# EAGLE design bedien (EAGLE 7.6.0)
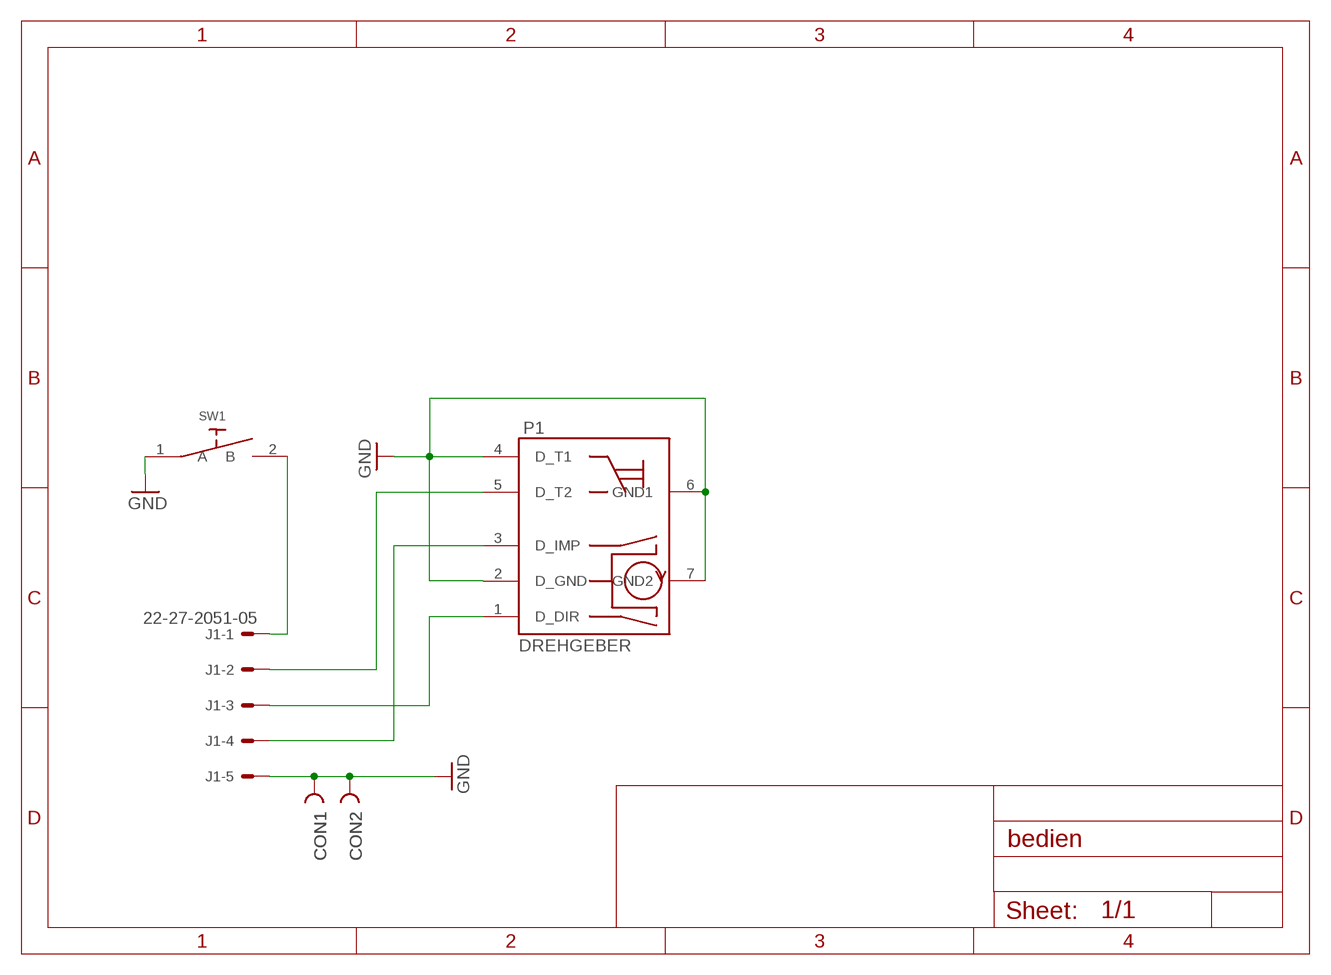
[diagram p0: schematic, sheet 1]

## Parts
CON1  PIN2_53MM  [HOLE3]
CON2  PIN2_53MM  [HOLE3]
J1  22-27-2051-05  [6410-05]
P1  DREHGEBER  [DREHG]
SW1  MTG-TASTER  [MTG]

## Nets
GND: CON1.1 CON2.1 J1.5 P1.2(D_GND) P1.4(D_T1) P1.6(GND1) P1.7(GND2) SW1.1(A)
N$1: J1.3 P1.1(D_DIR)
N$2: J1.4 P1.3(D_IMP)
N$3: J1.2 P1.5(D_T2)
N$4: J1.1 SW1.2(B)

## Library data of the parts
CON1 CON2 = lindenau:PIN2_5
J1 = con-molex:22-?-05: CONNECTOR wire to board 2.54 mm (.1 inch) pitch header; OC_FARNELL: unknown; OC_NEWARK: unknown
P1 = lindenau:DREHGEBER
SW1 = lindenau:MTG-TASTER

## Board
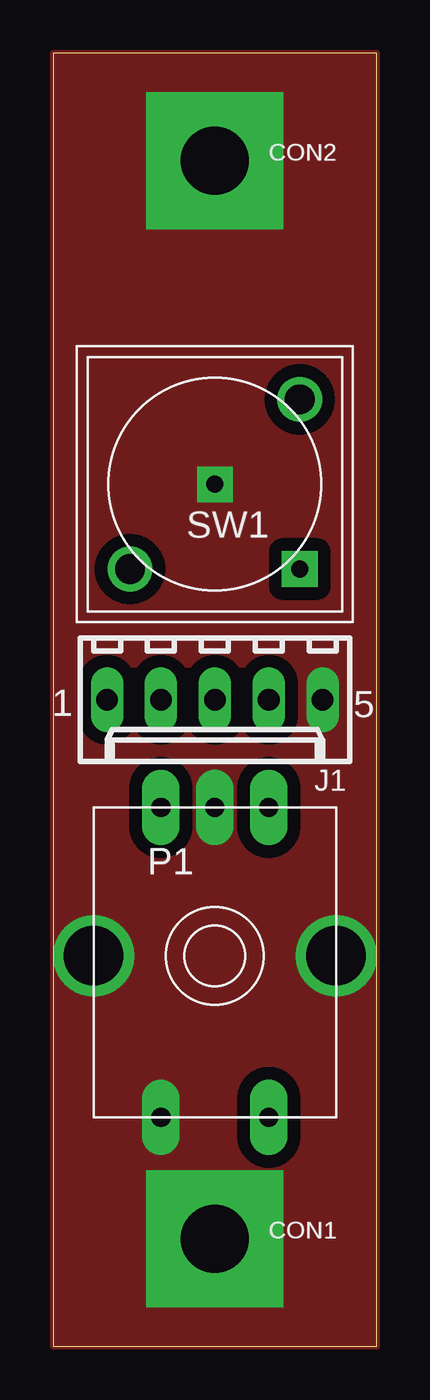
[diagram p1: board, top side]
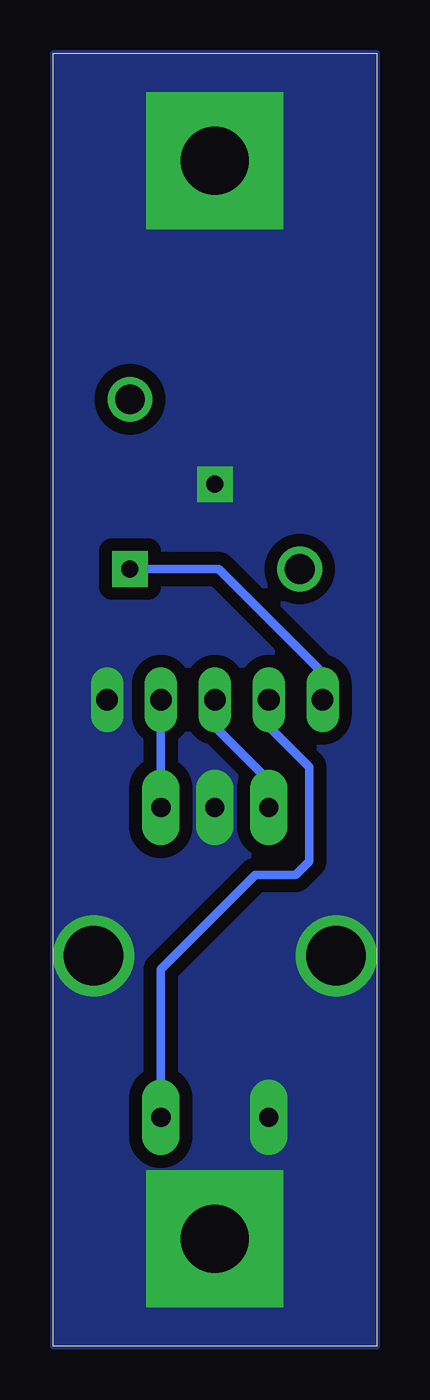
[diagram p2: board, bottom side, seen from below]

Size 15.24 x 60.96 mm. Coordinates in mm from the lower left corner, seen from the top.
Outline: 0,60.96 0,0 15.24,0 15.24,60.96 0,60.96
Copper layers (1*16): Top 0.035mm / dielectric 1.5mm / Bottom 0.035mm
Design rules "default *": minimum track width 10mil, minimum drill 24mil, track to track 8mil, track to pad 8mil, pad to pad 8mil, via to via 8mil, smd to smd 8mil, copper to edge 0mil, drill to drill 8mil, minimum pad ring 10mil, minimum via ring 8mil, stop-mask expansion 4mil, vias tented up to drill 0mil, thermal gap 10mil

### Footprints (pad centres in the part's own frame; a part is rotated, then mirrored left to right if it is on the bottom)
HOLE3 = drill 3.2 pad 6.452 square: 1 0,0
6410-05 = drill 1.016 long: 1 5.08,0; 2 2.54,0; 3 0,0; 4 -2.54,0; 5 -5.08,0
DREHG = drill 0.9 pad 1.778 long: 1 3.175,14.605; 2 5.715,14.605; 3 8.255,14.605; 4 3.175,0; 5 8.255,0 | drill 2.8: 6 0,7.62 | drill 2.8 pad 3.81: 7 11.43,7.62
MTG = drill 0.8 pad 1.676 square: 1 0,0; 2 -4,4 | drill 1.4: P$3 -4,-4; P$4 4,4

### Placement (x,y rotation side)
CON1  7.62,5.08 0 top
CON2  7.62,55.88 0 top
J1  7.62,30.48 180 top
P1  1.91,10.79 0 top
SW1  7.62,40.64 180 top

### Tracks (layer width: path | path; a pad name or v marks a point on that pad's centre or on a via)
GND
  pour Bottom (isolate 0.61, no thermals): 0,0 15.24,0 15.24,60.96 0,60.96
  pour Top (isolate 0.61, no thermals): 0,0 15.24,0 15.24,60.96 0,60.96
N$1
  Bottom 0.406: P1.1 5.08,26.67 7.62,29.21 J1.3
N$2
  Bottom 0.406: P1.3 J1.4
N$3
  Bottom 0.406: P1.5 10.16,17.78 5.71,22.23 3.81,22.23 3.17,22.86 3.17,27.3 5.08,29.21 J1.2
N$4
  Bottom 0.406: SW1.2 7.43,36.64 2.54,31.75 J1.1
